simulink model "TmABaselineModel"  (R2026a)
settings: Solver=ode1  StopTime=0.4  FixedStep=0.00001
libraries: LoomingNeuronLibrary x1

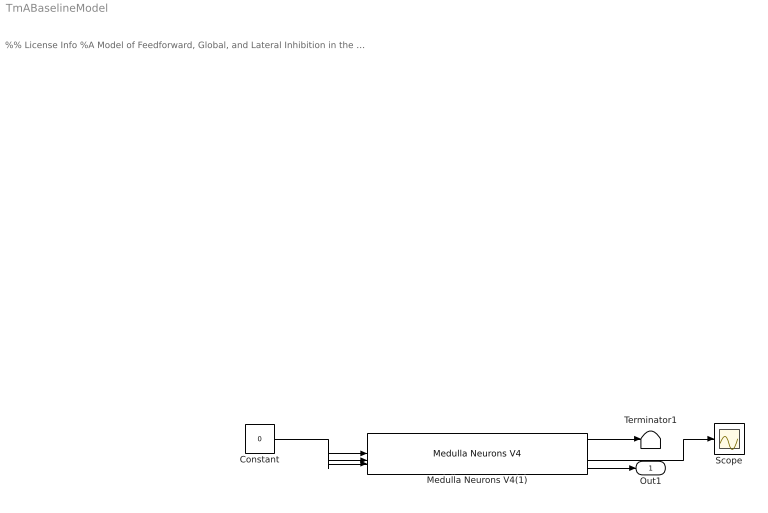
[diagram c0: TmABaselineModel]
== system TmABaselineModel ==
  note: %% License Info %A Model of Feedforward, Global, and Lateral Inhibition in the Locust Visual System. %This model examines the architecture and function of inhibitory mechanisms in the %visual system of locusts, namely those involved in the processing of inputs to a %key looming-sensitive neuron, the lobula giant movement detector (LGMD). %Copyright (c) 2026, Erik Olson, Travis Wiens, and Jack Gray %CITATION: %When using the model code for scientific publications, cite the following work: %Olson EGN, Wiens TK, Gray JR. A model of feedforward, global, and lateral inhibition %in the locust visual system predicts responses to looming stimuli. Biol Cybern. 2021 %Jun;115(3):245-265. doi: 10.1007/s00422-021-00876-8. Epub 2021 May 16. PMID: 33997912. %This program is free software: you can redistribute it and/or modify %it under the terms of the GNU General Public License as published by %the Free Software Foundation, either version 3 of the License, or %(at your option) any later version. %This program is distributed in the hope that it will be useful, %but WITHOUT ANY WARRANTY; without even the implied warranty of %MERCHANTABILITY or FITNESS FOR A PARTICULAR PURPOSE. See the %GNU General Public License for more details. %You should have received a copy of the GNU General Public License %along with this program. If not, see <https://www.gnu.org/licenses/>. %Contact: erik.olson@usask.ca
  Constant : Constant  Value=0
  Medulla Neurons V4(1) : LoomingNeuronLibrary/Medulla Neurons V4  K_in_ex=K_E_m  K_in_lateral=0  K_in_global=0  g_m=g_L_m  c_m=c  E_rev_ex=E_E  E_rev_inh=E_I  E_rest=E_L  V_t=V_t  Delta_t=Delta_t_m  V_fire=V_fire  tau=tau_alpha_m  g_med_adap_inc=Delta_g_A_m  tau_med_adap=tau_A_m  E_rev_adap=E_A  g_noise=g_N_m  noise_T=T_noise  radius=1
  Scope : Scope
  Terminator1 : Terminator
  Out1 : Outport
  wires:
  Constant/1 -> Medulla Neurons V4(1)/2, Medulla Neurons V4(1)/3, Medulla Neurons V4(1)/1
  Medulla Neurons V4(1)/1 -> Terminator1/1
  Medulla Neurons V4(1)/3 -> Out1/1
  Medulla Neurons V4(1)/2 -> Scope/1
